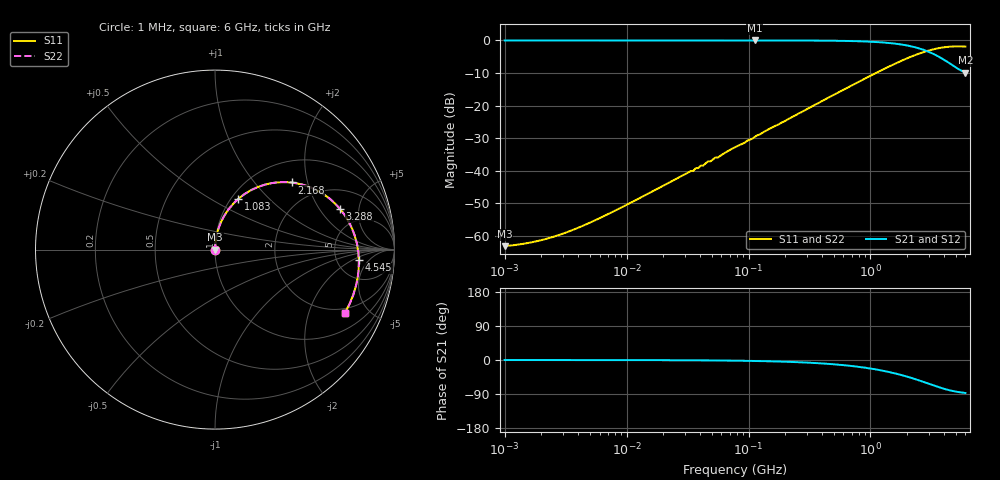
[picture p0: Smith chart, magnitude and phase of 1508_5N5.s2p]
# MHz S MA R 50
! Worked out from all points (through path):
!   189 points, 1 MHz to 6 GHz, reference 50 ohm
!   highest |S21| = -0.01 dB at 112.2 MHz (marker M1); lowest = -9.9 dB at 6 GHz (marker M2)
!   group delay of S21, straight-line fit = 49.7 ps
!   lowest |S11| = -63.1 dB at 1 MHz (marker M3), VSWR 1.00, Z = 50.1 + j0.0294 ohm
!   |S11| at or under -10 dB: start of sweep to 1.108 GHz
!   |S22| runs from -63.1 to -1.8 dB; largest |S21 - S12| = 0
!   S11 on the Smith chart (normalised r, x): 1 MHz: 1.00, +0.00; 1.083 GHz: 1.08, +0.67; 2.168 GHz: 1.45, +1.59; 3.288 GHz: 3.22, +3.15; 4.545 GHz: 8.24, -2.79; 6 GHz: 1.76, -3.52
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1  0.0006993 24.8  0.999 -0.0  0.999 -0.0  0.0006994 24.9
2.097  0.0008847 44.1  0.999 -0.0  0.999 -0.0  0.0008849 44.1
4.396  0.00144 63.8  0.999 -0.1  0.999 -0.1  0.001441 63.8
18.454  0.005463 82.9  0.999 -0.4  0.999 -0.4  0.005465 82.9
36.943  0.011 85.8  0.999 -0.8  0.999 -0.8  0.011 85.8
38.693  0.011 85.9  0.999 -0.9  0.999 -0.9  0.011 85.9
42.444  0.012 86.1  0.999 -1.0  0.999 -1.0  0.013 86.1
46.56  0.014 86.3  0.999 -1.1  0.999 -1.1  0.014 86.3
48.765  0.014 86.4  0.999 -1.1  0.999 -1.1  0.014 86.4
77.46  0.023 86.7  0.999 -1.8  0.999 -1.8  0.023 86.7
112.163  0.033 86.4  0.999 -2.5  0.999 -2.5  0.033 86.4
340.538  0.1 81.9  0.994 -7.7  0.994 -7.7  0.1 81.9
650.904  0.19 75.1  0.981 -14.7  0.981 -14.7  0.19 75.1
1082.877  0.31 65.4  0.949 -24.3  0.949 -24.3  0.31 65.4
1429.415  0.4 57.6  0.913 -31.9  0.913 -31.9  0.4 57.6
2167.84  0.567 41.3  0.81 -47.3  0.81 -47.3  0.567 41.3
2732.184  0.664 29.2  0.716 -57.9  0.716 -57.9  0.664 29.2
3287.73  0.732 18.1  0.62 -66.9  0.62 -66.9  0.732 18.1
3956.237  0.782 5.7  0.513 -75.4  0.513 -75.4  0.783 5.7
4545.398  0.804 -4.3  0.434 -80.7  0.434 -80.7  0.804 -4.3
5222.297  0.811 -14.8  0.367 -84.4  0.367 -84.4  0.811 -14.8
6000  0.805 -26.0  0.32 -87.1  0.32 -87.1  0.805 -26.0
